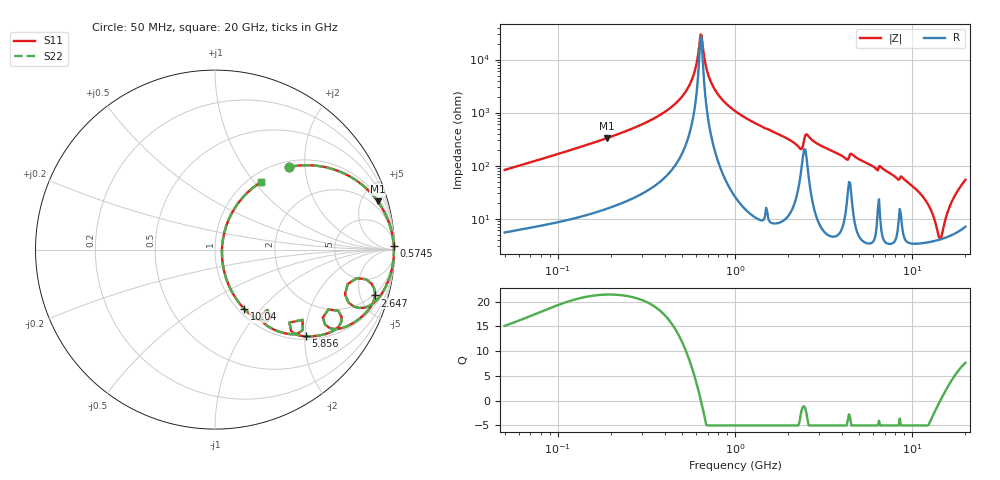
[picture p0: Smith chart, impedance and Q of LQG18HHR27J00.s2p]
!Murata Part Number: LQG18HHR27J00
!These Parameters are Measured in Series Mode Connection
!  o--[Z]--o
!Port1  Port2
!  o-------o
!Freq. Start=50[MHz] Stop=20[GHz], 401[Steps]
# Hz S RI R 50
!Freq.(Hz) S11(Real) S11(Imag) S21(Real) S21(Imag) S12(Real) S12(Imag) S22(Real) S22(Imag)
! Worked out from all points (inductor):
!   401 points, 50 MHz to 20 GHz, reference 50 ohm
!   read as one part in series: L = 259 nH near 51.52 MHz
!   highest Q = 21.4 at 189.6 MHz (marker M1), where L = 277 nH
!   self-resonance near 638 MHz
!   S11 on the Smith chart (normalised r, x): 50 MHz: 1.11, +1.65; 574.5 MHz: 15, +87; 2.647 GHz: 1.82, -6.62; 5.856 GHz: 1.07, -2.03; 10.04 GHz: 1.07, -0.82; 20 GHz: 1.14, +1.08
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5e7  0.4125 0.4603  0.5875 -0.4603  0.5875 -0.4603  0.4125 0.4603
1.364002e8  0.8283 0.3538  0.1717 -0.3538  0.1717 -0.3538  0.8283 0.3538
1.896393e8  0.9058 0.2697  0.0942 -0.2697  0.0942 -0.2697  0.9058 0.2697
3.721004e8  0.9813 0.111  0.0187 -0.111  0.0187 -0.111  0.9813 0.111
4.872511e8  0.9926 0.0552  0.0074 -0.0552  0.0074 -0.0552  0.9926 0.0552
5.745257e8  0.996 0.0222  0.004 -0.0222  0.004 -0.0222  0.996 0.0222
6.285508e8  0.9968 0.00429  0.00316 -0.00429  0.00316 -0.00429  0.9968 0.00429
6.476653e8  0.997 -0.0017  0.00304 0.0017  0.00304 0.0017  0.997 -0.0017
6.980337e8  0.9969 -0.0167  0.00308 0.0167  0.00308 0.0167  0.9969 -0.0167
7.523192e8  0.9964 -0.0319  0.00363 0.0319  0.00363 0.0319  0.9964 -0.0319
1e9  0.9892 -0.0921  0.0108 0.0921  0.0108 0.0921  0.9892 -0.0921
2.279204e9  0.8011 -0.3248  0.1989 0.3248  0.1989 0.3248  0.8011 -0.3248
2.493527e9  0.841 -0.1652  0.159 0.1652  0.159 0.1652  0.841 -0.1652
2.647493e9  0.891 -0.2557  0.109 0.2557  0.109 0.2557  0.891 -0.2557
2.728004e9  0.8846 -0.2846  0.1154 0.2846  0.1154 0.2846  0.8846 -0.2846
5.856089e9  0.5083 -0.4833  0.4917 0.4833  0.4917 0.4833  0.5083 -0.4833
7.442007e9  0.354 -0.4559  0.646 0.4559  0.646 0.4559  0.354 -0.4559
1.004137e10  0.1634 -0.3307  0.8366 0.3307  0.8366 0.3307  0.1634 -0.3307
1.238412e10  0.0616 -0.1592  0.9384 0.1592  0.9384 0.1592  0.0616 -0.1592
1.438523e10  0.0389 -0.00232  0.9611 0.00232  0.9611 0.00232  0.0389 -0.00232
1.670968e10  0.0797 0.1749  0.9203 -0.1749  0.9203 -0.1749  0.0797 0.1749
2e10  0.2539 0.3747  0.7461 -0.3747  0.7461 -0.3747  0.2539 0.3747
